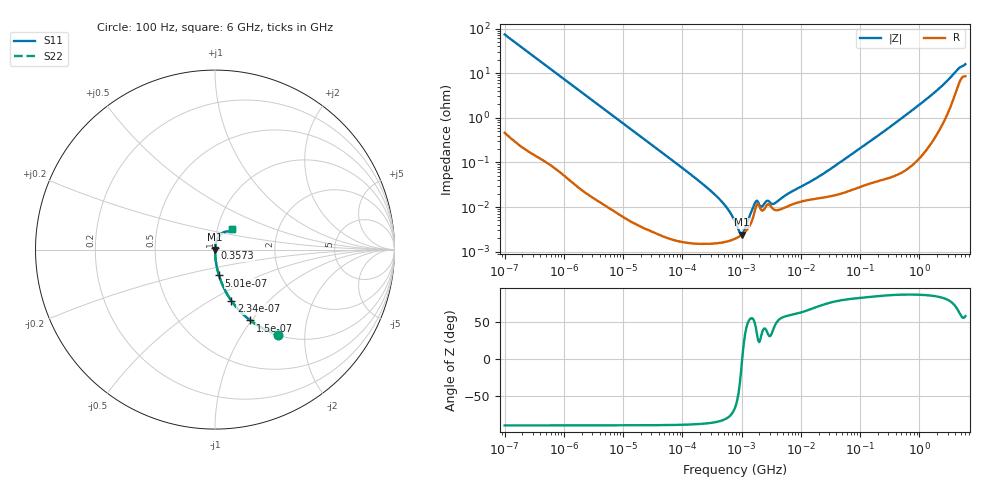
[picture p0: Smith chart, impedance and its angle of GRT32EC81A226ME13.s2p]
!Murata Part Number: GRT32EC81A226ME13
!These Parameters are Measured in Series Mode Connection
!Data Generated on Jun 19, 2026
!  o--ll--o
!Port1  Port2
!  o------o
!Operation Temp=25[degC], DC Bias Voltage=0[V]
!Freq. Start=100[Hz] Stop=6[GHz] 401[Steps]
# Hz S RI R 50
!Freq.(Hz) S11(Real) S11(Imag) S21(Real) S21(Imag) S12(Real) S12(Imag) S22(Real) S22(Imag)
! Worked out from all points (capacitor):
!   401 points, 100 Hz to 6 GHz, reference 50 ohm
!   read as one part in series: C = 21.6 uF near 109 Hz
!   lowest |Z| = 2.4 mohm at 1.013 MHz (marker M1)
!   series resonance near 1.024 MHz, so ESL is about 1.1 nH
!   S11 on the Smith chart (normalised r, x): 100 Hz: 1.01, -1.47; 150 Hz: 1.01, -0.99; 234 Hz: 1.00, -0.63; 501 Hz: 1.00, -0.30; 357.3 MHz: 1.00, +0.01; 6 GHz: 1.17, +0.27
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100  0.3523 -0.4746  0.6477 0.4746  0.6477 0.4746  0.3523 -0.4746
150  0.1967 -0.3946  0.8033 0.3946  0.8033 0.3946  0.1967 -0.3946
234  0.0918 -0.2858  0.9082 0.2858  0.9082 0.2858  0.0918 -0.2858
501  0.0223 -0.1442  0.9777 0.1442  0.9777 0.1442  0.0223 -0.1442
2008  0.00161 -0.037  0.9984 0.037  0.9984 0.037  0.00161 -0.037
40335  2.74e-05 -0.00187  1 0.00187  1 0.00187  2.74e-05 -0.00187
231233  1.5e-05 -0.000311  1 0.000311  1 0.000311  1.5e-05 -0.000311
541393  1.66e-05 -0.000102  1 0.000102  1 0.000102  1.66e-05 -0.000102
774597  1.94e-05 -4.33e-05  1 4.33e-05  1 4.33e-05  1.94e-05 -4.33e-05
1013323  2.39e-05 -1.7e-06  1 1.7e-06  1 1.7e-06  2.39e-05 -1.7e-06
1449809  4.42e-05 6.26e-05  1 -6.26e-05  1 -6.26e-05  4.42e-05 6.26e-05
1813585  0.000116 7.71e-05  0.9999 -7.71e-05  0.9999 -7.71e-05  0.000116 7.71e-05
2169299  8.47e-05 5.41e-05  0.9999 -5.41e-05  0.9999 -5.41e-05  8.47e-05 5.41e-05
2713602  0.000112 8.08e-05  0.9999 -8.08e-05  0.9999 -8.08e-05  0.000112 8.08e-05
3549919  8.72e-05 8.07e-05  0.9999 -8.07e-05  0.9999 -8.07e-05  8.72e-05 8.07e-05
6353432  0.000107 0.000176  0.9999 -0.000176  0.9999 -0.000176  0.000107 0.000176
1.555665e7  0.000149 0.000363  0.9999 -0.000363  0.9999 -0.000363  0.000149 0.000363
3.124326e8  0.000487 0.00606  0.9995 -0.00606  0.9995 -0.00606  0.000487 0.00606
3.573489e8  0.000527 0.00692  0.9995 -0.00692  0.9995 -0.00692  0.000527 0.00692
2.679998e9  0.0121 0.0572  0.9879 -0.0572  0.9879 -0.0572  0.0121 0.0572
4.385646e9  0.0548 0.099  0.9452 -0.099  0.9452 -0.099  0.0548 0.099
6e9  0.0926 0.1125  0.9074 -0.1125  0.9074 -0.1125  0.0926 0.1125
